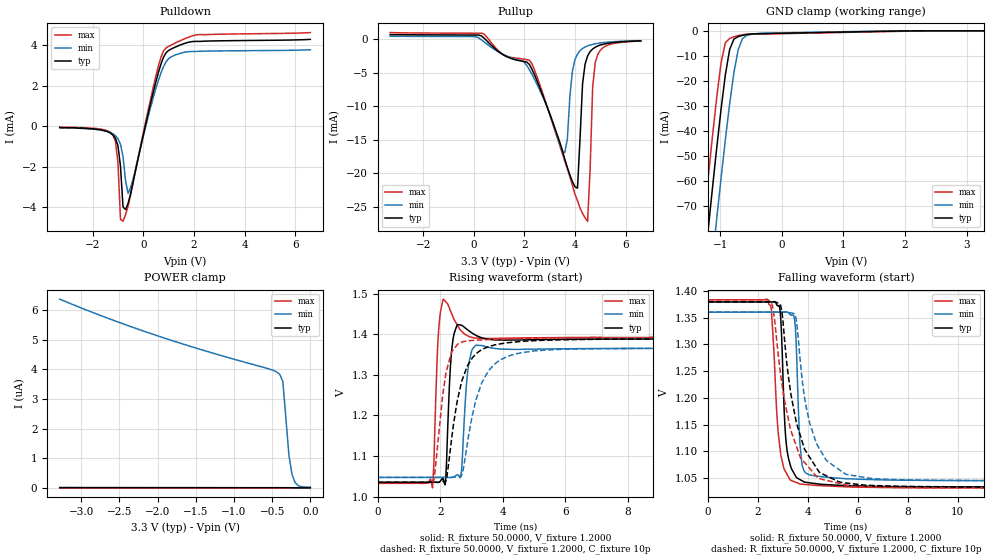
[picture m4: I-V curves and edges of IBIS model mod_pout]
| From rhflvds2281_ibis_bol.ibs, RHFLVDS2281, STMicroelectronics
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|   Model mod_pout
[Model]   mod_pout
Model_type 3-state
Polarity   Non-Inverting
Enable   Active-High
Vmeas  =   1.280V
Cref   =   10pF
C_comp   0.670pF   0.640pF   0.735pF
[Temperature Range]   25.0000   0.1250k   -55.0000
[Voltage Range]   3.3000V   3.0000V   3.6000V
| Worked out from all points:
|   slope of the pulldown table from 0 to 0.495 V, typ, clamps not added: 189 ohm
|   slope of the pullup table from 0 to 0.495 V, typ, clamps not added: 635 ohm
|   GND clamp passes 1 mA (typ) near -0.05 V on its own axis
|   rising waveform, R_fixture 50.0000, V_fixture 1.2000: 20-80 % time 112ps typ, 152ps min, 85.8ps max; typ from 1.03 V to 1.39 V
|   rising waveform, R_fixture 50.0000, V_fixture 1.2000, C_fixture 10p: 20-80 % time 540ps typ, 657ps min, 347ps max; typ from 1.03 V to 1.39 V
|   falling waveform, R_fixture 50.0000, V_fixture 1.2000: 20-80 % time 212ps typ, 160ps min, 287ps max; typ from 1.38 V to 1.03 V
|   falling waveform, R_fixture 50.0000, V_fixture 1.2000, C_fixture 10p: 20-80 % time 820ps typ, 782ps min, 856ps max; typ from 1.38 V to 1.03 V
[Pulldown]
|Voltage   I(typ)   I(min)   I(max)
-3.3V     -60uA      -70uA      -40uA
-1.2V     -426uA     -370uA     -431uA
-1.1V     -594uA     -462uA     -728uA
-1V       -953uA     -613uA     -1.784mA
-900mV    -1.969mA   -889uA     -4.592mA
-800mV    -3.985mA   -1.483mA   -4.695mA
-700mV    -4.113mA   -2.688mA   -4.37mA
-600mV    -3.813mA   -3.315mA   -3.95mA
500mV     2.207mA    1.874mA    2.487mA
900mV     3.636mA    3.189mA    3.875mA
2.2V      4.197mA    3.707mA    4.534mA
6.6V      4.298mA    3.785mA    4.633mA
[Pullup]
|Voltage   I(typ)   I(min)   I(max)
-3.3V     648.5uA    400.1uA    948.4uA
100mV     580uA      314.9uA    848.8uA
2.2V      -3.798mA   -4.575mA   -3.171mA
3.6V      -17.93mA   -16.93mA   -18.2mA
3.9V      -21.25mA   -4.76mA    -21.81mA
4.1V      -22.23mA   -2.252mA   -24.09mA
4.3V      -6.681mA   -1.42mA    -26mA
4.5V      -2.525mA   -1.04mA    -27.16mA
4.6V      -1.88mA    -910uA     -19.26mA
4.7V      -1.5mA     -810uA     -7.122mA
4.8V      -1.24mA    -720uA     -3.553mA
6.6V      -290uA     -260uA     -310uA
[GND_clamp]
|Voltage   I(typ)   I(min)   I(max)
-3.3V     -618mA     -644.4mA   -599.6mA
-1.27V    -96.79mA   -125.4mA   -76.01mA
-1.2V     -79.78mA   -108.4mA   -58.97mA
-1.06V    -46.87mA   -75.13mA   -26.67mA
-990mV    -31.49mA   -59.06mA   -12.94mA
-920mV    -17.71mA   -43.62mA   -4.778mA
-850mV    -7.485mA   -29.22mA   -3.049mA
-780mV    -3.3mA     -16.64mA   -2.381mA
-710mV    -2.307mA   -7.455mA   -1.88mA
-640mV    -1.824mA   -3.103mA   -1.539mA
-570mV    -1.491mA   -1.839mA   -1.352mA
3.28V     398.8pA    1.1uA      344.5pA
[POWER_clamp]
|Voltage   I(typ)   I(min)   I(max)
-3.28V    11.12nA    6.375uA    879.4pA
-2.68V    9.647nA    5.759uA    798.9pA
-2.04V    8.295nA    5.171uA    713.1pA
-560mV    5.839nA    4.032uA    514.6pA
-440mV    5.672nA    3.914uA    498.4pA
-400mV    5.615nA    3.831uA    492.8pA
-360mV    5.552nA    3.594uA    486.1pA
-280mV    5.327nA    1.1uA      469.9pA
-240mV    4.607nA    456.8nA    448.7pA
-200mV    1.988nA    184.6nA    409.6pA
-160mV    800.9pA    80.06nA    397.9pA
0V        401.5pA    24.41nA    379.3pA
[Ramp]
| variable   typ   min   max
dV/dt_r  0.2630/0.2424n   0.2113/0.3499n   0.3262/0.1812n
dV/dt_f  0.1093/71.0793p   0.1010/0.1209n   0.1112/69.1504p
R_load = 50.0000
[Rising Waveform]
R_fixture= 50.0000
V_fixture= 1.2000
V_fixture_min= 1.2000
V_fixture_max= 1.2000
|time   V(typ)   V(min)   V(max)
0s        1.035V     1.047V     1.033V
1.755ns   1.035V     1.047V     1.022V
1.92ns    1.035V     1.047V     1.37V
2.1ns     1.044V     1.047V     1.486V
2.175ns   1.04V      1.047V     1.48V
2.355ns   1.348V     1.047V     1.453V
2.55ns    1.424V     1.054V     1.422V
2.895ns   1.41V      1.316V     1.396V
3.135ns   1.398V     1.372V     1.391V
15ns      1.388V     1.365V     1.392V
[Rising Waveform]
R_fixture= 50.0000
V_fixture= 1.2000
V_fixture_min= 1.2000
V_fixture_max= 1.2000
C_fixture=10p
|time   V(typ)   V(min)   V(max)
0s        1.035V     1.047V     1.033V
1.755ns   1.035V     1.047V     1.032V
1.83ns    1.035V     1.047V     1.059V
2.19ns    1.039V     1.047V     1.306V
2.52ns    1.223V     1.049V     1.371V
2.73ns    1.293V     1.064V     1.382V
3.03ns    1.342V     1.2V       1.385V
3.33ns    1.362V     1.28V      1.386V
4.26ns    1.38V      1.348V     1.389V
15ns      1.388V     1.365V     1.392V
[Falling Waveform]
R_fixture= 50.0000
V_fixture= 1.2000
V_fixture_min= 1.2000
V_fixture_max= 1.2000
|time   V(typ)   V(min)   V(max)
0s        1.379V     1.36V      1.383V
2.505ns   1.379V     1.36V      1.373V
2.865ns   1.37V      1.36V      1.112V
2.94ns    1.321V     1.36V      1.087V
3.105ns   1.127V     1.361V     1.062V
3.315ns   1.07V      1.355V     1.046V
3.495ns   1.054V     1.332V     1.042V
3.675ns   1.047V     1.116V     1.039V
3.915ns   1.042V     1.059V     1.038V
15ns      1.033V     1.045V     1.032V
[Falling Waveform]
R_fixture= 50.0000
V_fixture= 1.2000
V_fixture_min= 1.2000
V_fixture_max= 1.2000
C_fixture=10p
|time   V(typ)   V(min)   V(max)
0s        1.379V     1.36V      1.383V
2.46ns    1.379V     1.36V      1.381V
2.64ns    1.379V     1.36V      1.355V
2.88ns    1.375V     1.36V      1.253V
3.51ns    1.16V      1.351V     1.113V
3.9ns     1.101V     1.19V      1.077V
4.41ns    1.064V     1.109V     1.049V
5.52ns    1.04V      1.057V     1.037V
6.57ns    1.036V     1.049V     1.033V
15ns      1.033V     1.045V     1.032V
